VAR_GLOBAL	
(* =========================== Acquisition Data , Data Block , Data Block Buffer =========================== *)
	AcquisitionData 				AT %I* : ARRAY [1..nMaxAcqNodeNo] OF stAcquisitionData;			(* Acquisition data from IO *)

	AcquisitionBlock				: ARRAY [1..nMaxAcqNodeNo] OF stAcquisitionBlock;		(*  Put one Acq Block into fifo buffer *)


	

(* ============================================ File Storge Path  ============================================ *)
	sFileTargetNetId	: T_AmsNetId := '';
	sAccessPath			: T_MaxString := 'C:\Data\';	//'\Hard Disk\ftp\'; 	(* Storge Folder Path *)


(* ===================================================================================================================== *)
	nRecordAcqBlockPerFile	: UDINT	:= 100;	(* File size = sizeof(file Header) + (sizeof(stAcquisitionData)* (nAcquisitionBlock+1) * nRecordAcqBlockPerFile   *)


END_VAR

VAR_GLOBAL CONSTANT
	nMaxAcqNodeNo		: UINT := 1;		(* IO Acquisition data node array , FirstId Start from 1  *) 
	nAcquisitionBlock	: UINT := 99;		(* Acquisition times to trig fifo buffer  , Don't less then 20 (reserve for handshake process)    *)
	nFifoSize			: UINT := 10;		(* Define Buffer size *)
END_VAR
